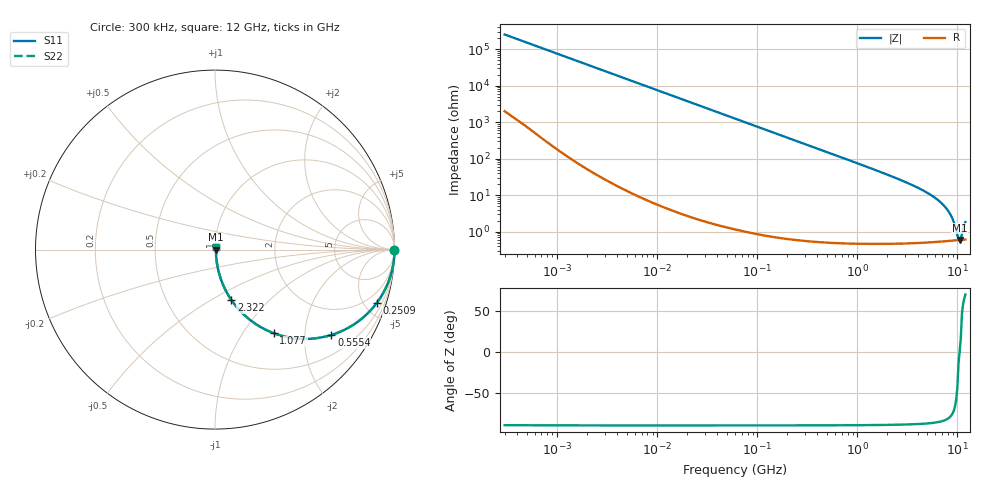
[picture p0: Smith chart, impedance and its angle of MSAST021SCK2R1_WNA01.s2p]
! MSAST021SCK2R1_WNA01  S-PARAMETER MODEL  ( General Type )
! Model Generated by TAIYO YUDEN Corporation (http://www.ty-top.com)
! Version 2.0
! TAIYO YUDEN Control No. 181101
! Copyright(c) 2015 TAIYO YUDEN CO.,LTD. All Rights Reserved.
! Product Description (link to TY-COMPAS)
! https://ds.yuden.co.jp/TYCOMPAS/or/detail?pn=MSAST021SCK2R1BWNA01&u=M
! Products Name : Multilayer Ceramic Capacitors
! Characteristics :
!  Capacitance : 2.1 pF , Rated Voltage : 25V , TCC : CK / C0K
!  Case Size : 0.25 x 0.125 / 0.0098 x 0.0049 [mm/inch] , Thickness : 0.125 / 0.0049 [mm/inch]
!  (Conditions: Temperature = 25 degC , DC Bias Current/Voltage = 0A / 0V)
! External Node Assignments :
!  1  o---| |---o  2
! GND o---------o GND
! Frequency Range : 0.3MHz  -  12000MHz  [ 401 STEP ]
# MHz S RI R 50
! Freq[MHz].  S11 Real  S11 Imag  S21 Real  S21 Imag  S12 Real  S12 Imag  S22 Real  S22 Imag
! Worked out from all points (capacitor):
!   401 points, 300 kHz to 12 GHz, reference 50 ohm
!   read as one part in series: C = 2.1 pF near 316.3 kHz
!   lowest |Z| = 593 mohm at 10.51 GHz (marker M1)
!   series resonance near 10.49 GHz, so ESL is about 110 pH
!   S11 on the Smith chart (normalised r, x): 300 kHz: open; 250.9 MHz: 1.01, -6.04; 555.4 MHz: 1.01, -2.72; 1.077 GHz: 1.01, -1.39; 2.322 GHz: 1.01, -0.62; 12 GHz: 1.01, +0.03
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0.3  1 -0.000396  3.29e-06 0.000396  3.29e-06 0.000396  1 -0.000396
1.769972  1 -0.00234  8.91e-06 0.00234  8.91e-06 0.00234  1 -0.00234
10.44266  0.9998 -0.0138  0.0002 0.0138  0.0002 0.0138  0.9998 -0.0138
60  0.9937 -0.0787  0.0063 0.0787  0.0063 0.0787  0.9937 -0.0787
125.9782  0.9729 -0.1617  0.0271 0.1617  0.0271 0.1617  0.9729 -0.1617
250.8588  0.9007 -0.2981  0.0993 0.2981  0.0993 0.2981  0.9007 -0.2981
353.9943  0.8199 -0.383  0.1801 0.383  0.1801 0.383  0.8199 -0.383
555.3718  0.6488 -0.4755  0.3512 0.4755  0.3512 0.4755  0.6488 -0.4755
763.2128  0.4938 -0.4976  0.5062 0.4976  0.5062 0.4976  0.4938 -0.4976
1076.992  0.3275 -0.466  0.6725 0.466  0.6725 0.466  0.3275 -0.466
2088.533  0.1113 -0.3079  0.8887 0.3079  0.8887 0.3079  0.1113 -0.3079
2321.999  0.0912 -0.2804  0.9088 0.2804  0.9088 0.2804  0.0912 -0.2804
4385.161  0.0244 -0.1377  0.9756 0.1377  0.9756 0.1377  0.0244 -0.1377
6699.894  0.00956 -0.0648  0.9904 0.0648  0.9904 0.0648  0.00956 -0.0648
7648.807  0.00746 -0.0445  0.9925 0.0445  0.9925 0.0445  0.00746 -0.0445
8503.825  0.00643 -0.0287  0.9936 0.0287  0.9936 0.0287  0.00643 -0.0287
9207.246  0.006 -0.0171  0.994 0.0171  0.994 0.0171  0.006 -0.0171
9968.853  0.00585 -0.00559  0.9942 0.00559  0.9942 0.00559  0.00585 -0.00559
10236.47  0.00586 -0.00153  0.9941 0.00153  0.9941 0.00153  0.00586 -0.00153
10511.28  0.00589 0.000141  0.9941 -0.000141  0.9941 -0.000141  0.00589 0.000141
10793.46  0.00593 0.00175  0.9941 -0.00175  0.9941 -0.00175  0.00593 0.00175
12000  0.00638 0.0172  0.9936 -0.0172  0.9936 -0.0172  0.00638 0.0172
